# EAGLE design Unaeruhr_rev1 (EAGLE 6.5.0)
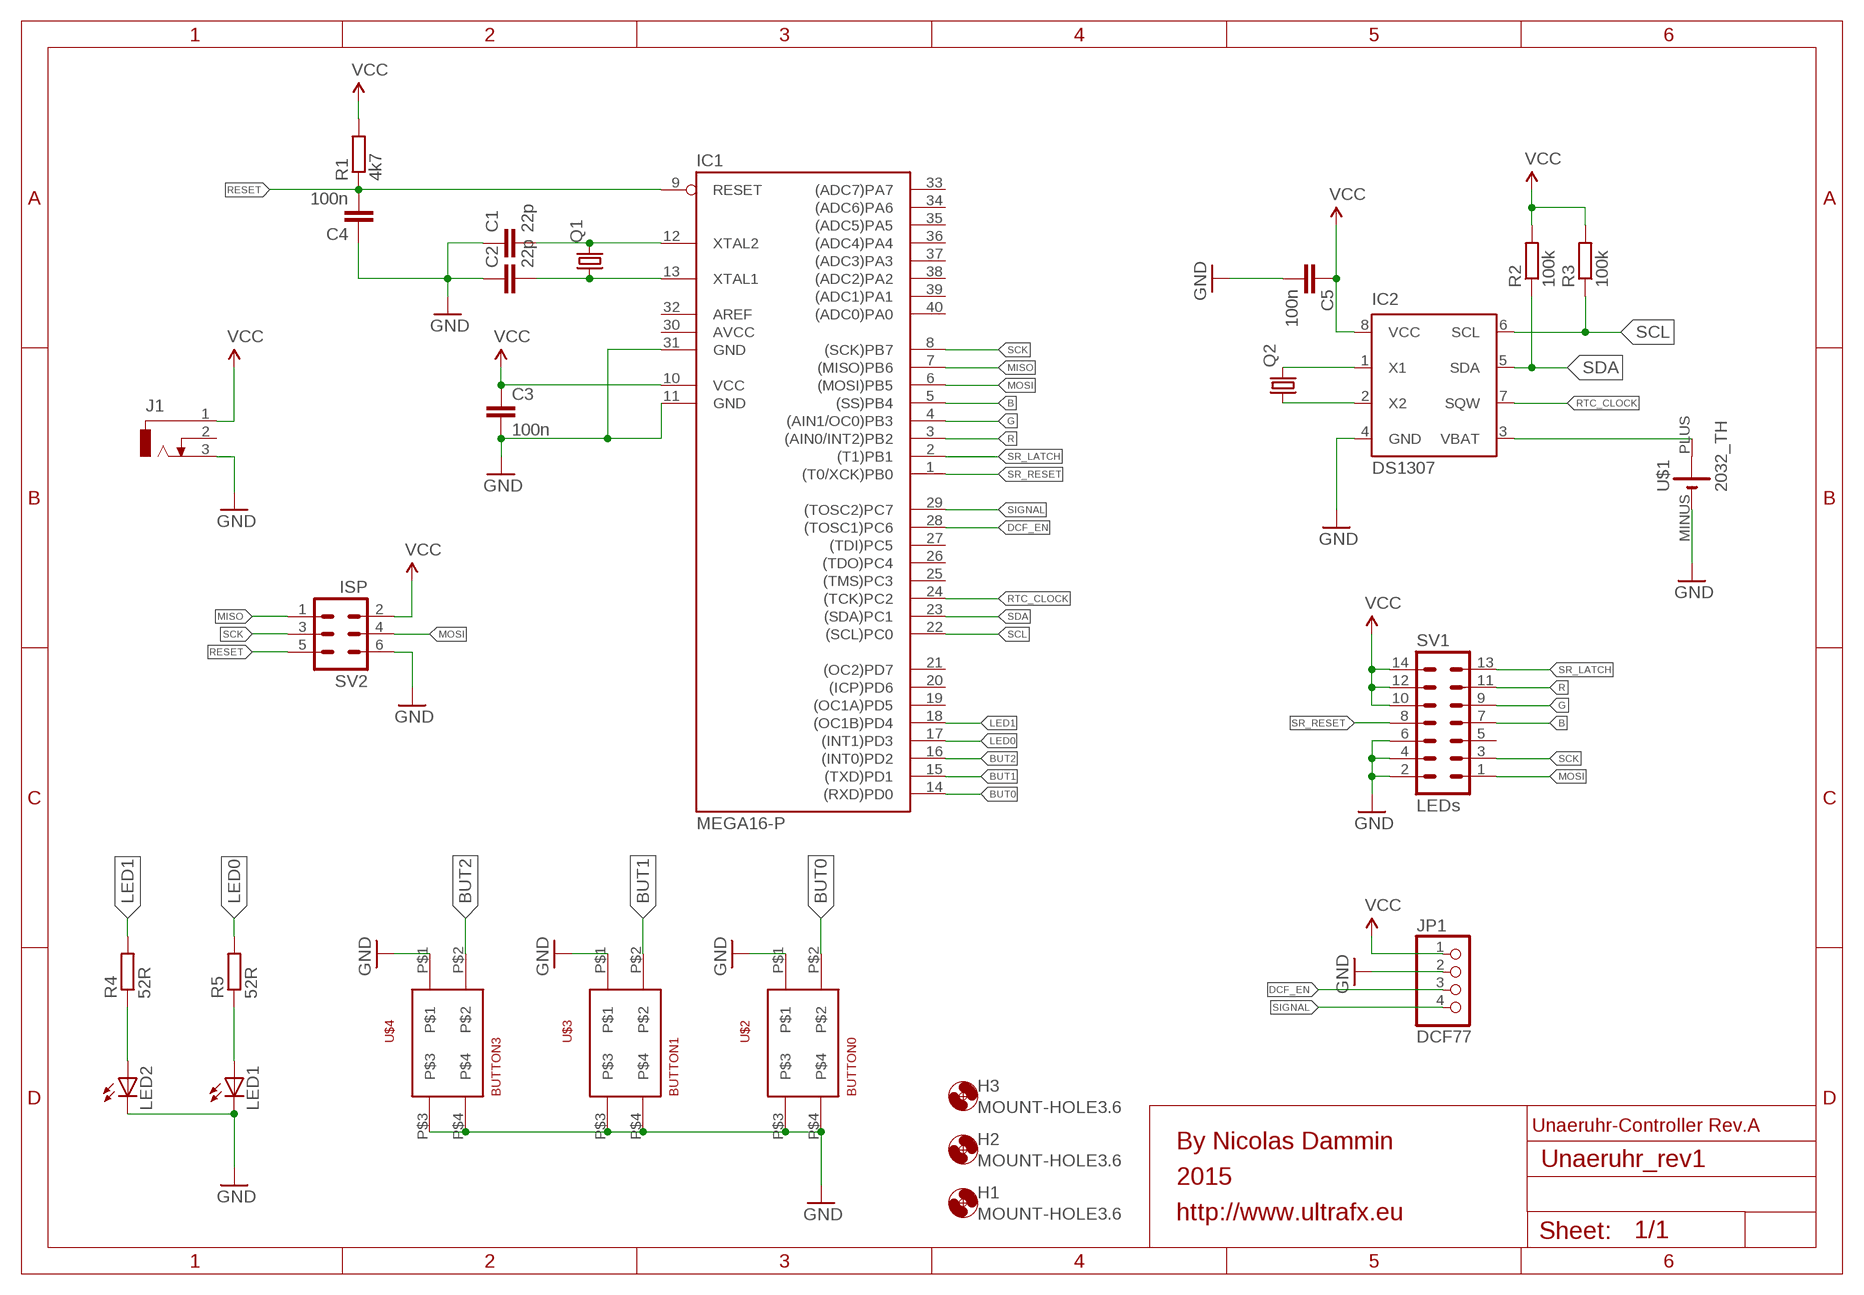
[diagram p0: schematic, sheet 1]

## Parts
C1  22p  C-EUC0805  [C0805]
C2  22p  C-EUC0805  [C0805]
C3  100n  C-EUC0805  [C0805]
C4  100n  C-EUC0805  [C0805]
C5  100n  C-EUC0805  [C0805]
H1  MOUNT-HOLE3.6  [3,6]
H2  MOUNT-HOLE3.6  [3,6]
H3  MOUNT-HOLE3.6  [3,6]
IC1  MEGA16-P  [DIL40]
IC2  DS1307  [DIL08]
J1  DCJ0303  [DCJ0303]
JP1  DCF77  PINHD-1X4  [1X04]
LED1  LED5MM  [LED5MM]
LED2  LED5MM  [LED5MM]
Q1  CRYSTALHC49S  [HC49/S]
Q2  CRYSTALTC38H  [TC38H]
R1  4k7  R-EU_R0805  [R0805]
R2  100k  R-EU_R0805  [R0805]
R3  100k  R-EU_R0805  [R0805]
R4  52R  R-EU_R0805  [R0805]
R5  52R  R-EU_R0805  [R0805]
SV1  LEDs  ML14  [ML14]
SV2  ISP  ML6  [ML6]
U$1  2032_TH  [KZH20]
U$2  BUTTON0  TASTER3305  [3305]
U$3  BUTTON1  TASTER3305  [3305]
U$4  BUTTON3  TASTER3305  [3305]

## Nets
B: IC1.5((SS)PB4) SV1.7
BUT0: IC1.14((RXD)PD0) U$2.P$2
BUT1: IC1.15((TXD)PD1) U$3.P$2
BUT2: IC1.16((INT0)PD2) U$4.P$2
DCF_EN: IC1.28((TOSC1)PC6) JP1.3
G: IC1.4((AIN1/OC0)PB3) SV1.9
GND: C1.1 C2.1 C3.2 C4.1 C5.2 IC1.11(GND) IC1.31(GND) IC2.4(GND) J1.3 JP1.2 LED1.K(C) LED2.K(C) SV1.2 SV1.4 SV1.6 SV2.6 U$1.MINUS(-) U$2.P$1 U$2.P$3 U$2.P$4 U$3.P$1 U$3.P$3 U$3.P$4 U$4.P$1 U$4.P$3 U$4.P$4
LED0: IC1.17((INT1)PD3) R5.2
LED1: IC1.18((OC1B)PD4) R4.2
MISO: IC1.7((MISO)PB6) SV2.1
MOSI: IC1.6((MOSI)PB5) SV1.1 SV2.4
N$3: C1.2 IC1.12(XTAL2) Q1.2
N$4: C2.2 IC1.13(XTAL1) Q1.1
N$5: LED2.A R4.1
N$6: LED1.A R5.1
N$9: IC2.3(VBAT) U$1.PLUS(+)
N$12: IC2.1(X1) Q2.2
N$13: IC2.2(X2) Q2.1
R: IC1.3((AIN0/INT2)PB2) SV1.11
RESET: C4.2 IC1.9(RESET) R1.1 SV2.5
RTC_CLOCK: IC1.24((TCK)PC2) IC2.7(SQW)
SCK: IC1.8((SCK)PB7) SV1.3 SV2.3
SCL: IC1.22((SCL)PC0) IC2.6(SCL) R3.1
SDA: IC1.23((SDA)PC1) IC2.5(SDA) R2.1
SIGNAL: IC1.29((TOSC2)PC7) JP1.4
SR_LATCH: IC1.2((T1)PB1) SV1.13
SR_RESET: IC1.1((T0/XCK)PB0) SV1.8
VCC: C3.1 C5.1 IC1.10(VCC) IC2.8(VCC) J1.1 JP1.1 R1.2 R2.2 R3.2 SV1.10 SV1.12 SV1.14 SV2.2
Unconnected: IC1.19((OC1A)PD5) IC1.20((ICP)PD6) IC1.21((OC2)PD7) IC1.25((TMS)PC3) IC1.26((TDO)PC4) IC1.27((TDI)PC5) IC1.32(AREF) IC1.33((ADC7)PA7) IC1.34((ADC6)PA6) IC1.35((ADC5)PA5) IC1.36((ADC4)PA4) IC1.37((ADC3)PA3) IC1.38((ADC2)PA2) IC1.39((ADC1)PA1) IC1.40((ADC0)PA0) J1.2 SV1.5

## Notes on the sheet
- Unaeruhr-Controller Rev.A
- By Nicolas Dammin
- 2015
- http://www.ultrafx.eu

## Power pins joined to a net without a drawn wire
AVCC: IC1.30(AVCC)

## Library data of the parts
C1-C5 = rcl:C-EU: CAPACITOR, European symbol
H1-H3 = holes:MOUNT-HOLE: MOUNTING HOLE with drill center marker
IC1 = atmel:MEGA16-P: MICROCONTROLLER 16 Kbytes FLASH 1 kbytes SRAM 512 bytes EEPROM USART 8-channel 10 bit ADC Source: avr.lbr; MPN: ATMEGA16-16PU; OC_FARNELL: 9171142; OC_NEWARK: 01M6885
IC2 = ds1307_pcf8583:DS1307: I2C-Bus CLOCK/CALENDAR
J1 = con-jack:DCJ0303: DC POWER JACK Source: DCJ0303.pdf; OC_FARNELL: unknown; OC_NEWARK: unknown
JP1 = pinhead:PINHD-1X4: PIN HEADER
LED1 LED2 = led:LED: LED
Q1 = crystal:CRYSTAL: CRYSTAL; OC_FARNELL: 1667008; OC_NEWARK: unknown
Q2 = crystal:CRYSTAL: CRYSTAL; OC_FARNELL: unknown; OC_NEWARK: unknown
R1-R5 = rcl:R-EU_: RESISTOR, European symbol
SV1 = con-ml:ML14: HARTING; OC_FARNELL: unknown; OC_NEWARK: unknown
SV2 = con-ml:ML6: HARTING; OC_FARNELL: unknown; OC_NEWARK: unknown
U$1 = kzh20_lithium_batterie_holder:2032_TH
U$2-U$4 = TASTER_3305:TASTER3305

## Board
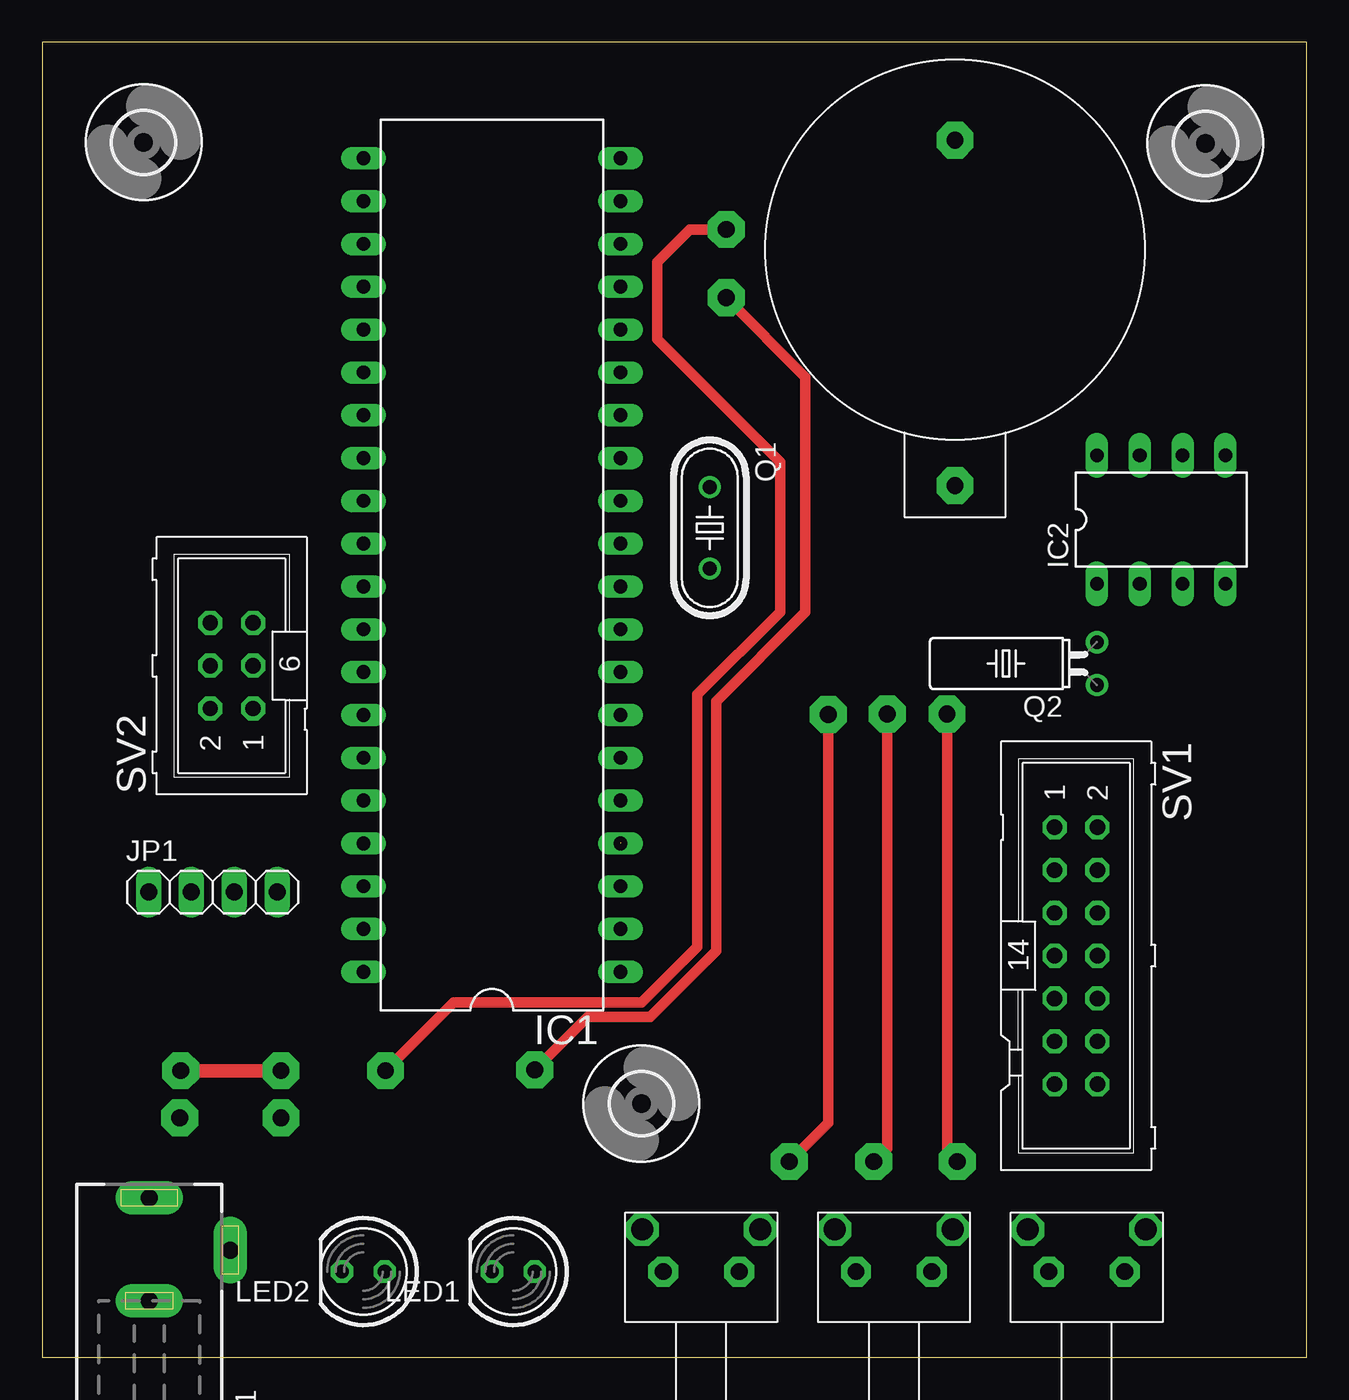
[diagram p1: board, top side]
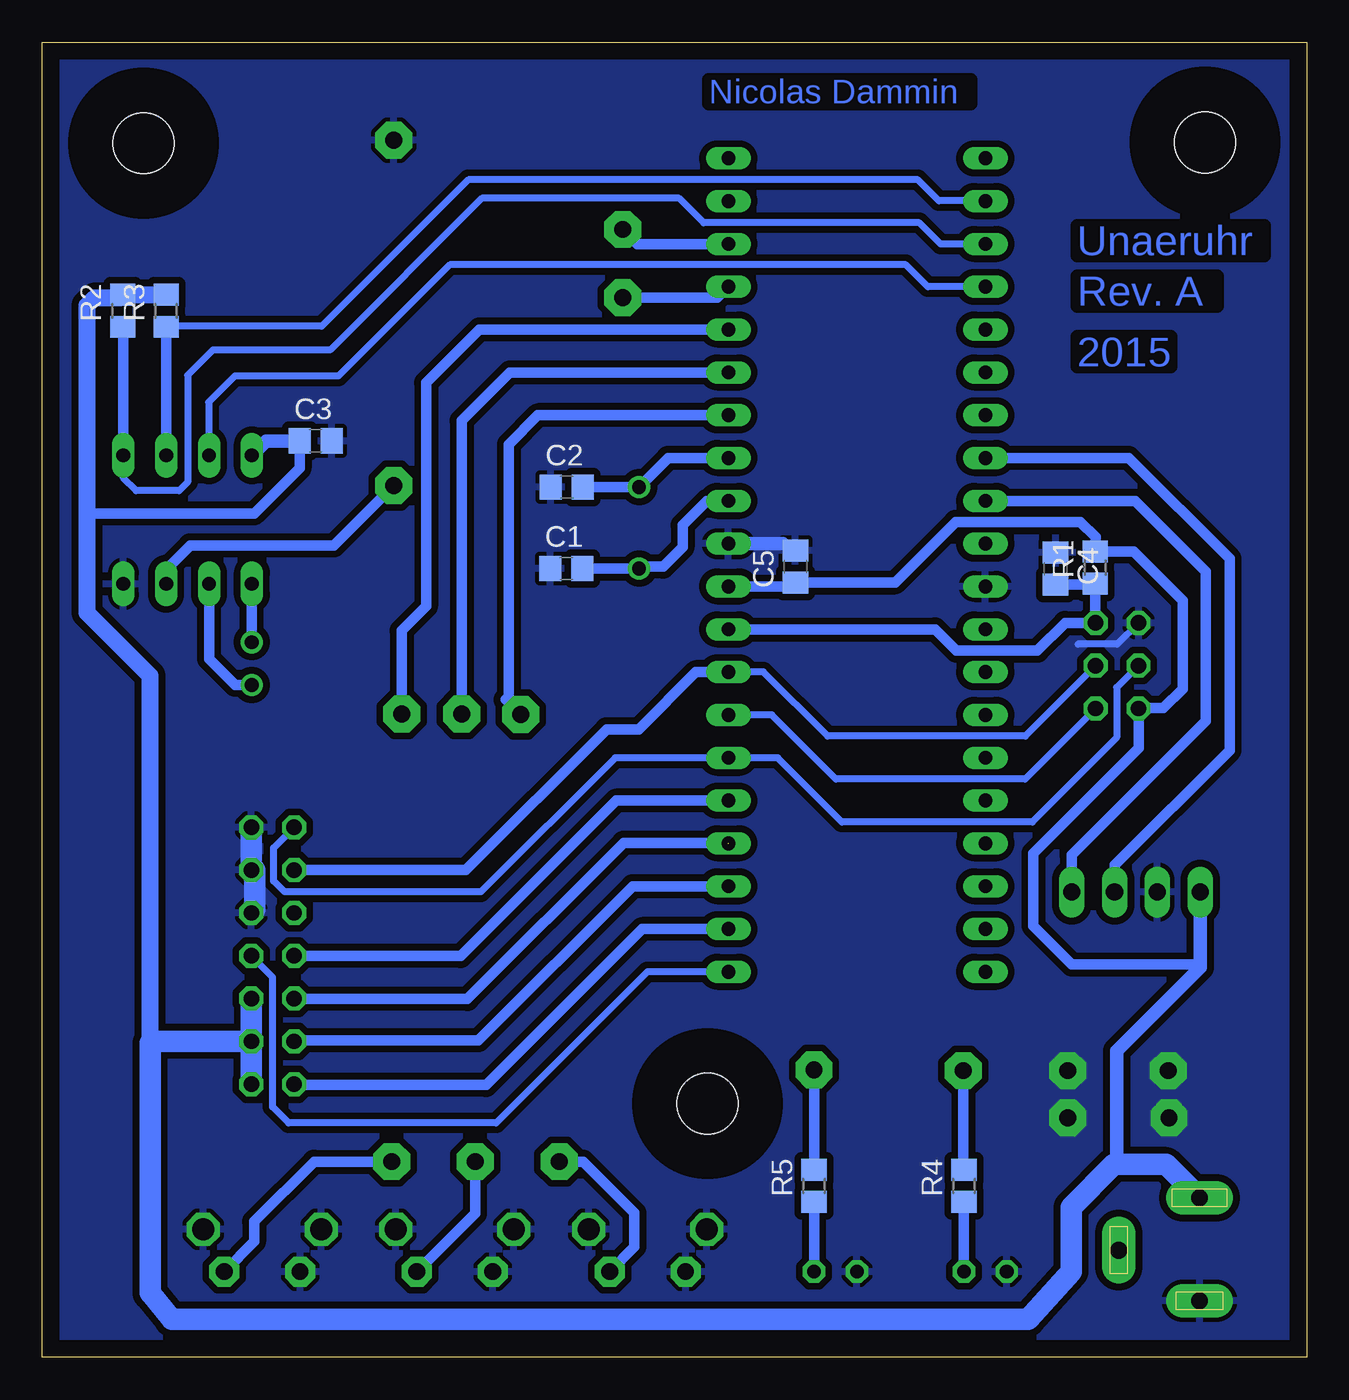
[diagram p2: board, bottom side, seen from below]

Size 74.98 x 78.02 mm. Coordinates in mm from the lower left corner, seen from the top.
Outline: 0,0.01 74.98,0 74.98,78.01 0,78.02 0,0.01
Copper layers (1*16): Top 0.035mm / dielectric 1.5mm / Bottom 0.035mm
Design rules "default *": minimum track width 10mil, minimum drill 24mil, track to track 6mil, track to pad 6mil, pad to pad 6mil, via to via 6mil, smd to smd 6mil, copper to edge 40mil, drill to drill 8mil, minimum pad ring 10mil, minimum via ring 8mil, stop-mask expansion 4mil, vias tented up to drill 0mil, thermal gap 10mil

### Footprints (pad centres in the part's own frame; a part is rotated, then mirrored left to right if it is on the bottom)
C0805 = smd 1.3 x 1.5: 1 -0.95,0; 2 0.95,0
3,6 = hole 3.6: 0,0
DIL40 = drill 0.813 long: 1 -24.13,-7.62; 2 -21.59,-7.62; 3 -19.05,-7.62; 4 -16.51,-7.62; 5 -13.97,-7.62; 6 -11.43,-7.62; 7 -8.89,-7.62; 8 -6.35,-7.62; 9 -3.81,-7.62; 10 -1.27,-7.62; 11 1.27,-7.62; 12 3.81,-7.62; 13 6.35,-7.62; 14 8.89,-7.62; 15 11.43,-7.62; 16 13.97,-7.62; 17 16.51,-7.62; 18 19.05,-7.62; 19 21.59,-7.62; 20 24.13,-7.62; 21 24.13,7.62; 22 21.59,7.62; 23 19.05,7.62; 24 16.51,7.62; 25 13.97,7.62; 26 11.43,7.62; 27 8.89,7.62; 28 6.35,7.62; 29 3.81,7.62; 30 1.27,7.62; 31 -1.27,7.62; 32 -3.81,7.62; 33 -6.35,7.62; 34 -8.89,7.62; 35 -11.43,7.62; 36 -13.97,7.62; 37 -16.51,7.62; 38 -19.05,7.62; 39 -21.59,7.62; 40 -24.13,7.62
DIL08 = drill 0.813 long: 1 -3.81,-3.81; 2 -1.27,-3.81; 3 1.27,-3.81; 4 3.81,-3.81; 5 3.81,3.81; 6 1.27,3.81; 7 -1.27,3.81; 8 -3.81,3.81
DCJ0303 = drill 1 pad 2 long: 1 0,3.1; 2 4.8,0; 3 0,-3
1X04 = drill 1.016 long: 1 -3.81,0; 2 -1.27,0; 3 1.27,0; 4 3.81,0
LED5MM = drill 0.813 octagon: A -1.27,0; K 1.27,0
HC49/S = drill 0.813: 1 -2.413,0; 2 2.413,0
TC38H = drill 0.813: 1 -1.27,0; 2 1.27,0
R0805 = smd 1.3 x 1.5: 1 -0.95,0; 2 0.95,0
ML14 = drill 0.914 octagon: 1 -7.62,-1.27; 2 -7.62,1.27; 3 -5.08,-1.27; 4 -5.08,1.27; 5 -2.54,-1.27; 6 -2.54,1.27; 7 0,-1.27; 8 0,1.27; 9 2.54,-1.27; 10 2.54,1.27; 11 5.08,-1.27; 12 5.08,1.27; 13 7.62,-1.27; 14 7.62,1.27
ML6 = drill 0.914 octagon: 1 -2.54,-1.27; 2 -2.54,1.27; 3 0,-1.27; 4 0,1.27; 5 2.54,-1.27; 6 2.54,1.27
KZH20 = drill 1 pad 2.184 octagon: MINUS 0,0; PLUS -20.5,0
3305 = drill 1 pad 1.778 octagon: P$1 0,0; P$2 4.5,0 | drill 1.3 pad 1.778 octagon: P$3 -1.25,2.5; P$4 5.75,2.5

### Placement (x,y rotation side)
C1  43.91,46.79 0 bottom
C2  43.87,51.62 0 bottom
C3  58.77,54.37 0 bottom
C4  14.89,46.8 270 bottom
C5  30.31,46.91 90 bottom
H1  6.02,72.08 0 top
H2  68.98,72.02 0 top
H3  35.53,15.05 0 top
IC1  26.67,47 90 top
IC2  66.36,49.7 0 top
J1  6.35,6.36 0 top
JP1  10.12,27.6 0 top
LED1  27.94,5.09 180 top
LED2  19.05,5.09 180 top
Q1  39.59,49.21 270 top
Q2  62.55,41.16 90 top
R1  12.54,46.85 90 bottom
R2  70.2,62.08 90 bottom
R3  67.63,62.08 90 bottom
R4  20.32,10.17 90 bottom
R5  29.21,10.17 90 bottom
SV1  61.31,23.82 270 top
SV2  11.24,41.03 90 top
U$1  54.13,72.21 90 top
U$2  36.83,5.09 0 top
U$3  48.26,5.09 0 top
U$4  59.69,5.09 0 top

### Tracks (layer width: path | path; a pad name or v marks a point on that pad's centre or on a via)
B
  Bottom 0.61: IC1.5 40.94,33.03 50.16,23.81 60.03,23.81 SV1.7
BUT0  (via drill 1 pad 2.18)
  Top 0.61: v46.61,38.14 46.61,13.91 v44.31,11.61
  Bottom 0.61: v46.61,38.14 47.5,39.02 47.31,39.21 47.31,54.16 45.58,55.89 IC1.14 | v44.31,11.61 42.91,11.61 39.86,8.56 39.86,6.56 U$2.P$2
BUT1  (via drill 1 pad 2.18)
  Top 0.61: v50.11,38.16 50.11,12.41 v49.31,11.61
  Bottom 0.61: 50.13,38.18 v50.11,38.16 50.11,55.56 47.24,58.43 IC1.15 | U$3.P$2 49.31,8.54 v49.31,11.61
BUT2  (via drill 1 pad 2.18)
  Top 0.61: v53.66,38.16 53.66,12.21 v54.26,11.61
  Bottom 0.61: U$4.P$2 62.41,6.87 62.41,8.06 58.86,11.61 v54.26,11.61 | IC1.16 49.05,60.97 52.21,57.81 52.21,44.56 53.66,43.11 v53.66,38.16
DCF_EN
  Bottom 0.61: IC1.28 10.55,53.35 4.57,47.37 4.57,36.01 11.39,29.2 JP1.3
G  (1 unrouted)
  Bottom 0.61: 34.32,30.52 40.5,30.52 49.76,21.26 60.02,21.26 SV1.9
GND  (via drill 1 pad 2.18)
  Top 0.813: v8.21,17.01 v14.16,17.01
  Bottom 0.406: 13.56,42.31 11.23,42.31 SV2.6
  Bottom 0.813: IC1.11 31.07,48.27
  Bottom 1.27: SV1.2 SV1.4 62.39,28.9 62.39,26.55 SV1.6
  other vias: 8.16,14.21 14.16,14.21
  pour Bottom (isolate 0.406): -0.19,78.66 75.01,78.66 75.01,-0.19 -0.19,-0.19 -0.19,78.61
LED0  (via drill 1 pad 2.18)
  Top 0.61: v29.21,17.06 32.36,20.21 36.06,20.21 39.96,24.11 39.96,38.91 45.26,44.21 45.26,58.16 v40.56,62.86
  Bottom 0.61: v29.21,17.06 R5.2 | IC1.17 34.94,62.86 v40.56,62.86
LED1  (via drill 1 pad 2.18)
  Top 0.61: v40.56,66.91 38.41,66.91 36.46,64.96 36.46,60.41 43.76,53.11 43.76,44.21 38.86,39.31 38.86,24.36 35.56,21.06 24.41,21.06 v20.36,17.01
  Bottom 0.61: IC1.18 39.7,66.05 v40.56,66.91 | v20.36,17.01 20.36,11.16 R4.2
MISO
  Bottom 0.406: SV2.1 16.69,34.31 27.91,34.31 31.71,38.11 IC1.7
MOSI
  Bottom 0.406: SV1.1 61.26,30.22 61.26,28.26 60.61,27.61 48.96,27.61 41,35.57 IC1.6 31.36,35.56 27.56,31.76 16.26,31.76 11.26,36.76 11.26,39.74 SV2.4
N$3
  Bottom 0.61: C1.2 Q1.2 39.47,46.91 38.16,46.91 37.01,48.06 37.01,49.36 35.56,50.81 IC1.12
N$4
  Bottom 0.61: C2.2 Q1.1 37.86,53.35 IC1.13
N$5
  Bottom 0.61: LED2.A R4.1
N$6
  Bottom 0.61: LED1.A R5.1
N$9
  Bottom 0.61: U$1.PLUS 57.68,48.16 66.21,48.16 67.63,46.74 IC2.3
N$12
  Bottom 0.61: Q2.2 IC2.1
N$13
  Bottom 0.61: Q2.1 63.54,39.89 65.09,41.44 IC2.2
R
  Bottom 0.61: IC1.3 39.97,27.95 49.11,18.81 59.97,18.81 SV1.11
RESET
  Bottom 0.61: IC1.9 22.04,43.19 20.77,41.92 15.97,41.92 14.32,43.57 SV2.5 12.54,43.6 R1.1 12.59,45.85 C4.2
RTC_CLOCK
  Bottom 0.406: IC1.24 22.46,63.51 23.76,64.81 50.81,64.81 57.41,58.21 63.56,58.21 65.11,56.66 65.11,53.53 IC2.7
SCK
  Bottom 0.406: SV2.3 16.68,36.86 28.41,36.86 32.21,40.66 IC1.8
  Bottom 0.61: SV1.3 49.86,28.91 41.51,37.26 39.61,37.26 36.22,40.65 IC1.8
SCL
  Bottom 0.406: IC1.22 19.07,68.61 21.81,68.61 23.06,69.86 49.71,69.86 58.41,61.16 67.6,61.16 R3.1
  Bottom 0.61: R3.1 IC2.6
SDA
  Bottom 0.406: IC1.23 21.7,66.05 22.96,67.31 35.76,67.31 37.21,68.76 48.91,68.76 57.91,59.76 64.86,59.76 66.36,58.26 66.36,51.91 66.86,51.41 69.41,51.41 70.17,52.17 IC2.5
  Bottom 0.61: 70.17,61.1 IC2.5
  Bottom 1.016: 70.17,61.1 R2.1
SIGNAL
  Bottom 0.61: IC1.29 10.16,50.81 5.97,46.62 5.97,37.75 13.93,29.79 JP1.4
SR_LATCH
  Bottom 0.61: IC1.2 39.41,25.41 48.66,16.16 60,16.16 SV1.13
SR_RESET
  Bottom 0.406: IC1.1 39.1,22.87 48.06,13.91 60.36,13.91 61.31,14.86 61.31,22.55 SV1.8
VCC
  Bottom 0.406: R1.2 12.54,47.99
  Bottom 0.61: C3.1 59.72,52.75 62.41,50.06 72.31,50.06 | 68.43,34.06 68.58,34.21 | IC1.10 30.55,45.73 C5.1 24.41,45.96 20.81,49.56 13.41,49.56 12.51,48.66 12.51,47.83 R1.2 10.25,47.8 7.36,44.91 7.36,39.66 8.51,38.51 9.95,38.51 SV2.2 9.97,36.14 16.21,29.9 16.21,25.59 13.93,23.31 6.31,23.31
  Bottom 0.813: IC2.8 61.69,54.37 C3.1 | 11.26,11.44 11.26,18.17 6.31,23.12 6.31,23.31 JP1.1
  Bottom 1.016: 68.58,18.65 68.58,34.21 68.58,40.43 72.31,44.16 72.31,50.06 72.31,62.41 71.86,62.86 70.37,62.86 R2.2 R3.2
  Bottom 1.27: J1.1 8.33,11.44 11.26,11.44 11.43,11.44 13.97,8.9 13.97,5.09 16.51,2.25 67.31,2.25 68.58,3.82 68.58,18.65 68.48,18.74 SV1.12 | SV1.14 SV1.12 | SV1.10 SV1.12

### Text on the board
Bottom: Nicolas Dammin | Unaeruhr | Rev. A | 2015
